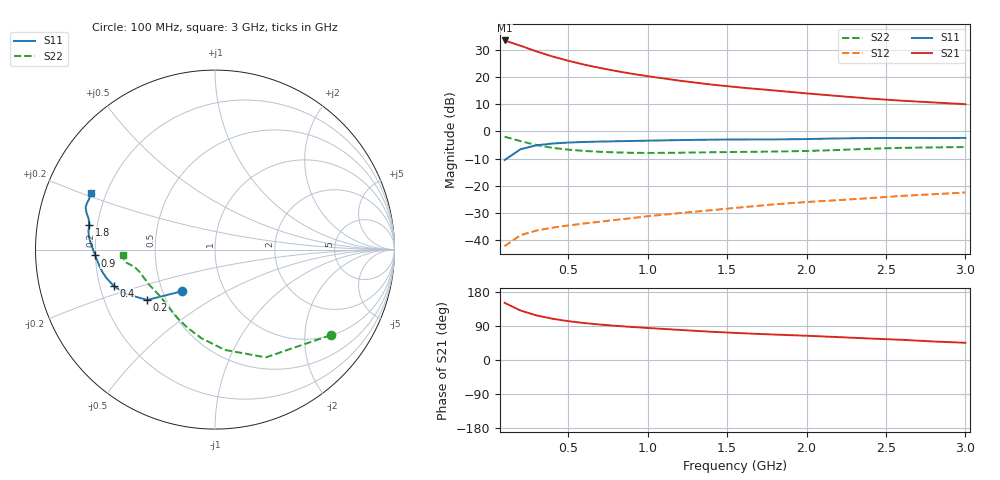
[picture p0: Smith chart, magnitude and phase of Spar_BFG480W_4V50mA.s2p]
! Filename: 450BFG480.001
! Title: BFG480W
! Bias: Vce=4V; Ic=50mA
! Company: NXP Semiconductors NL
! User: Quality&Reliability T&D
! Measure time: 10 Nov 1999 / 12:02:59
#  MHz  S  MA  R 50
! Freq  S11  S21  S12  S22  :
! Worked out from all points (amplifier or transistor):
!   20 points, 100 MHz to 3 GHz, reference 50 ohm
!   highest |S21| = 33.7 dB at 100 MHz (marker M1)
!   |S21| within 3 dB of that: start of sweep to 250.3 MHz
!   unconditionally stable (mu >= 1): 954.9 MHz to end of sweep
!   at 400 MHz: K = 0.65, MSG = 31.7 dB, |S12| = -35.6 dB
!   at 1.2 GHz: K = 1.05, MAG = 23.1 dB, |S12| = -30.2 dB
!   at 3 GHz: K = 1.06, MAG = 14.9 dB, |S12| = -22.6 dB
!   S11 on the Smith chart (normalised r, x): 100 MHz: 0.63, -0.32; 200 MHz: 0.39, -0.28; 400 MHz: 0.26, -0.16; 900 MHz: 0.20, -0.02; 1.8 GHz: 0.17, +0.10; 3 GHz: 0.14, +0.21
100  0.2968 -128.5  48.15 150.9  0.007593 66.1  0.8017 -36.5
200  0.4707 -143.4  38.43 130.6  0.01211 56.3  0.6639 -64.8
300  0.5549 -153.6  30.28 117.7  0.01474 53.0  0.5613 -84.5
400  0.5987 -160.2  24.43 108.9  0.01667 52.5  0.4994 -98.8
500  0.6243 -165.1  20.31 102.5  0.01831 53.6  0.4617 -109.4
600  0.6402 -168.9  17.24 97.6  0.01989 55.3  0.4376 -117.6
700  0.651 -172.1  14.95 93.6  0.02154 57.2  0.4215 -124.0
800  0.6597 -174.8  13.14 90.1  0.02324 59.3  0.4107 -129.4
900  0.668 -177.2  11.69 87.2  0.02503 61.6  0.4042 -134.1
1000  0.6768 -179.4  10.52 84.5  0.02712 63.2  0.4013 -138.3
1200  0.6934 177.0  8.702 79.5  0.031 66.0  0.4049 -145.2
1400  0.7061 174.2  7.378 74.6  0.03505 68.0  0.4135 -150.5
1600  0.7126 171.6  6.436 70.6  0.0399 69.7  0.4194 -154.4
1800  0.714 168.8  5.722 67.1  0.04512 71.1  0.4258 -158.4
2000  0.7246 166.3  5.064 64.0  0.04968 72.4  0.4361 -163.1
2200  0.7447 164.0  4.522 60.4  0.05389 72.9  0.4548 -167.2
2400  0.7575 162.1  4.057 56.7  0.05865 72.8  0.4794 -169.9
2600  0.7595 160.4  3.709 53.3  0.06456 72.6  0.4989 -171.6
2800  0.7559 158.1  3.442 48.9  0.06931 71.6  0.5083 -173.6
3000  0.7611 155.4  3.196 45.4  0.07455 71.1  0.516 -176.6
